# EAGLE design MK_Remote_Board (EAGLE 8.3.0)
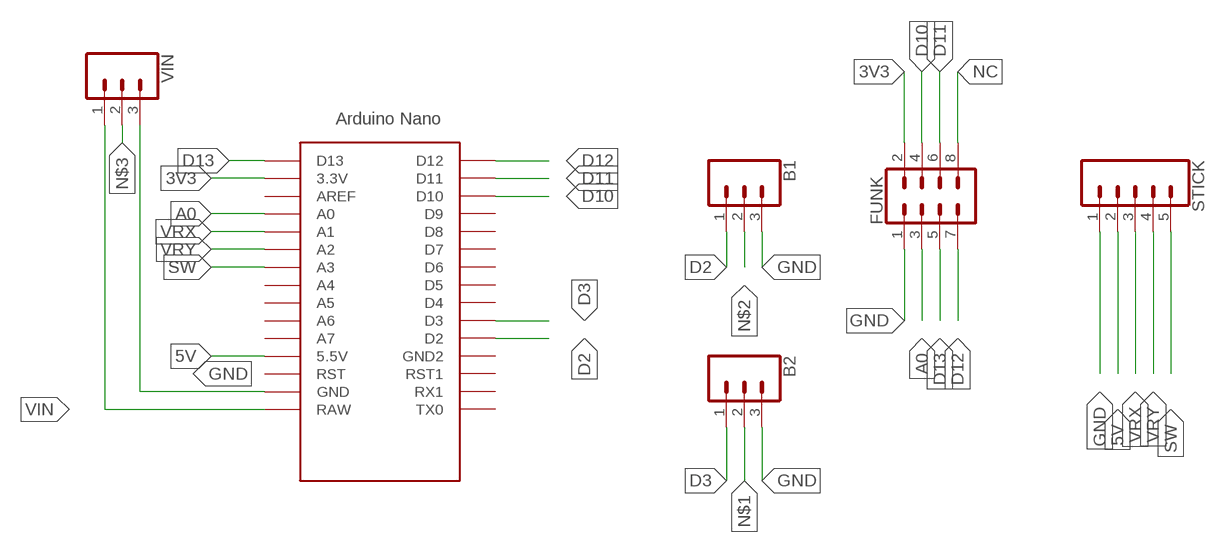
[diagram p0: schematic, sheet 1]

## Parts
B1  CONN_03  [1X03]
B2  CONN_03  [1X03]
FUNK  CONN_04X2  [2X4]
STICK  CONN_05  [1X05]
U$1  NANO  [NANO]
VIN  CONN_03  [1X03]

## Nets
3V3: FUNK.2 U$1.3.3V
5V: STICK.2 U$1.5V(5.5V)
A0: FUNK.3 U$1.A0
D2: B1.1 U$1.D2
D3: B2.1 U$1.D3
D10: FUNK.4 U$1.D10
D11: FUNK.6 U$1.D11
D12: FUNK.7 U$1.D12
D13: FUNK.5 U$1.D13
GND: B1.3 B2.3 FUNK.1 STICK.1 U$1.GND VIN.3
N$1: B2.2
N$2: B1.2
N$3: VIN.2
NC: FUNK.8
SW: STICK.5 U$1.A3
VIN: U$1.RAW VIN.1
VRX: STICK.3 U$1.A1
VRY: STICK.4 U$1.A2
Unconnected: U$1.A4 U$1.A5 U$1.A6 U$1.A7 U$1.AREF U$1.D4 U$1.D5 U$1.D6 U$1.D7 U$1.D8 U$1.D9 U$1.GND1(GND2) U$1.ICSP1 U$1.ICSP2 U$1.ICSP3 U$1.ICSP4 U$1.ICSP5 U$1.ICSP6 U$1.RST U$1.RST1 U$1.RX1 U$1.TX0

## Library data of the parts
B1 B2 VIN = SparkFun-Connectors:CONN_03: Multi connection point. Often used as Generic Header-pin footprint for 0.1 inch spaced/style header connections On any of the 0.1 inch spaced packages, you can populate with these: Break Away Headers - Straight (PRT-00116) Break Away Male Headers - Right Angle (PRT-00553) Female Headers (PRT-00115)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
FUNK = SparkFun-Connectors:CONN_04X2: Multi connection point. Often used as Generic Header-pin footprint for 0.1 inch spaced/style header connections On any of the 0.1 inch spaced packages, you can populate with these: Break Away Headers - Straight (PRT-00116) Break Away Male Headers - Right Angle (PRT-00553) Female Headers (PRT-00115)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
STICK = SparkFun-Connectors:CONN_05: Multi connection point. Often used as Generic Header-pin footprint for 0.1 inch spaced/style header connections On any of the 0.1 inch spaced packages, you can populate with these: Break Away Headers - Straight (PRT-00116) Break Away Male Headers - Right Angle (PRT-00553) Female Headers (PRT-00115)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
U$1 = Arduino-clone:NANO: Arduino Nano

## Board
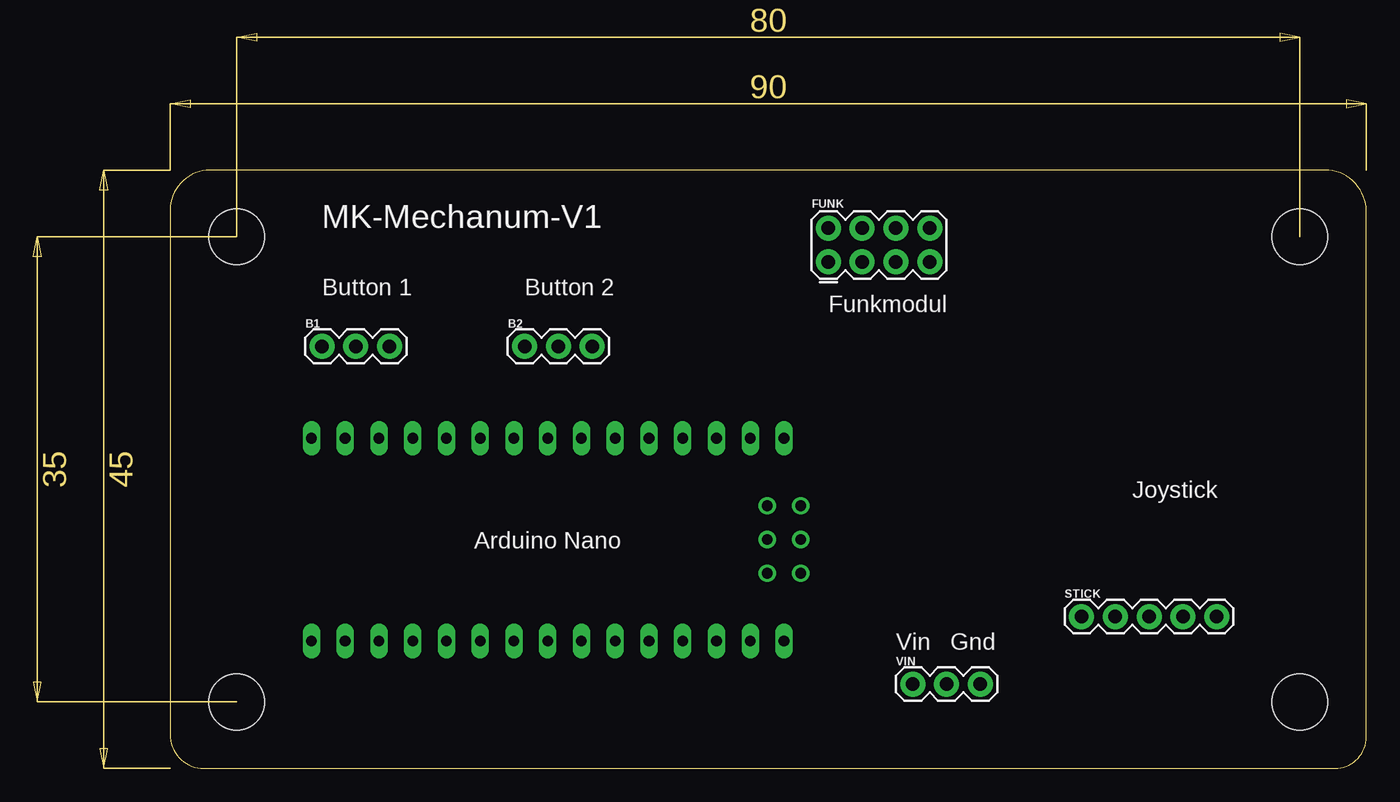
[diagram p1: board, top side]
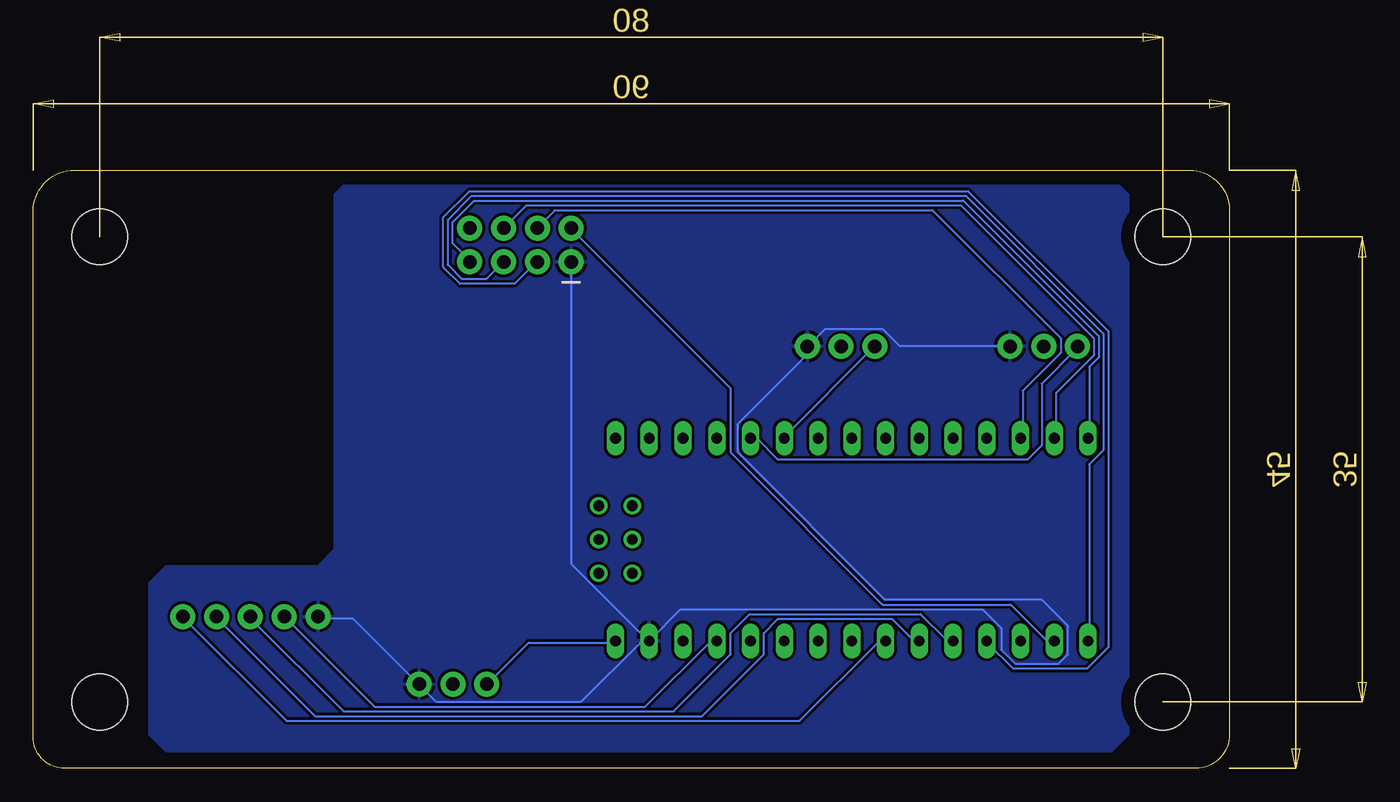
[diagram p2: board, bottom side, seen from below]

Size 100.3 x 55.3 mm. Coordinates in mm from the lower left corner, seen from the top.
Outline: 97.21,45 13.3,45 arc90 10.3,42 10.3,2.54 arc90 12.84,0 97.93,0 arc90 100.3,2.37 100.3,41.91 arc90 97.21,45
Copper layers (1*16): Top 0.035mm / dielectric 1.5mm / Bottom 0.035mm
Design rules "PCBway": minimum track width 6mil, minimum drill 0.3mm, track to track 0.205mm, track to pad 0.205mm, pad to pad 0.205mm, via to via 0.205mm, smd to smd 8mil, copper to edge 40mil, drill to drill 8mil, minimum pad ring 10mil, minimum via ring 8mil, stop-mask expansion 4mil, vias tented up to drill 25mil, thermal gap 10mil
Holes 4.2 mm at 15.3,40 15.3,5 95.3,40 95.3,5

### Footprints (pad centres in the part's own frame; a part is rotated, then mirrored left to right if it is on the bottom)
1X03 = drill 1.016 pad 1.88: 1 0,0; 2 2.54,0; 3 5.08,0
2X4 = drill 1.016 pad 1.88: 1 -3.81,-1.27; 2 -3.81,1.27; 3 -1.27,-1.27; 4 -1.27,1.27; 5 1.27,-1.27; 6 1.27,1.27; 7 3.81,-1.27; 8 3.81,1.27
1X05 = drill 1.016 pad 1.88: 1 0,0; 2 2.54,0; 3 5.08,0; 4 7.62,0; 5 10.16,0
NANO = drill 0.8 long: 3.3V -10.16,24.13; 5V -10.16,-1.27; A0 -10.16,19.05; A1 -10.16,16.51; A2 -10.16,13.97; A3 -10.16,11.43; A4 -10.16,8.89; A5 -10.16,6.35; A6 -10.16,3.81; A7 -10.16,1.27; AREF -10.16,21.59; D2 5.08,1.27; D3 5.08,3.81; D4 5.08,6.35; D5 5.08,8.89; D6 5.08,11.43; D7 5.08,13.97; D8 5.08,16.51; D9 5.08,19.05; D10 5.08,21.59; D11 5.08,24.13; D12 5.08,26.67; D13 -10.16,26.67; GND -10.16,-6.35; GND1 5.08,-1.27; RAW -10.16,-8.89; RST -10.16,-3.81; RST1 5.08,-3.81; RX1 5.08,-6.35; TX0 5.08,-8.89 | drill 0.8: ICSP1 -5.08,-10.16; ICSP2 -5.08,-7.62; ICSP3 -2.54,-10.16; ICSP4 -2.54,-7.62; ICSP5 0,-10.16; ICSP6 0,-7.62

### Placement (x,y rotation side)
B1  21.73,31.75 0 top
B2  36.97,31.75 0 top
FUNK  63.64,39.37 0 top
STICK  78.88,11.43 0 top
U$1  47.6,19.76 90 top
VIN  66.18,6.35 0 top

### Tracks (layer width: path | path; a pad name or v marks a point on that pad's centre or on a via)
3V3
  Bottom 0.152: U$1.3.3V 23.52,9.65 24.06,9.65 26.74,12.33 36.39,12.33 47.83,23.77 47.83,28.59 59.8,40.56 FUNK.2
5V
  Bottom 0.152: U$1.5V 48.9,9.47 49.44,9.47 54.26,4.65 74.63,4.65 81.24,11.26 STICK.2
A0
  Bottom 0.152: U$1.A0 28.53,9.47 26.56,7.5 21.02,7.5 19.41,9.11 19.41,32.88 29.96,43.42 67.48,43.42 69.45,41.46 69.45,37.71 68.2,36.45 64.09,36.45 62.48,38.06 FUNK.3
D2
  Bottom 0.152: U$1.D2 46.22,24.84 45.86,24.84 44.25,23.23 25.49,23.23 24.42,24.3 24.42,28.95 21.74,31.63 B1.1
D3
  Bottom 0.152: U$1.D3 43.72,25.02 37.11,31.63 B2.1
D10
  Bottom 0.152: U$1.D10 25.85,25.02 25.85,28.41 22.99,31.27 22.99,32.34 32.64,41.99 61.05,41.99 62.3,40.74 FUNK.4
D11
  Bottom 0.152: U$1.D11 23.34,25.02 23.34,28.23 20.49,31.09 20.49,32.34 30.49,42.35 63.2,42.35 64.8,40.74 FUNK.6
D12
  Bottom 0.152: U$1.D12 20.84,25.02 20.84,30.2 20.13,30.91 20.13,32.52 30.31,42.71 67.13,42.71 68.73,41.1 68.73,39.49 67.48,38.24 FUNK.7
D13
  Bottom 0.152: U$1.D13 20.84,9.65 20.84,22.87 19.77,23.95 19.77,32.7 30.14,43.07 67.31,43.07 69.09,41.28 69.09,37.88 68.02,36.81 66.23,36.81 64.98,38.06 FUNK.5
GND
  Bottom 0.152: B1.3 26.92,31.81 35.14,31.81 36.39,33.06 40.68,33.06 41.93,31.81 B2.3 42.11,31.63 42.11,31.09 47.29,25.91 47.29,23.77 36.21,12.69 24.42,12.69 22.45,10.72 22.45,8.58 23.17,7.86 26.38,7.86 27.46,8.94 27.46,10.54 28.89,11.97 51.58,11.97 53.9,9.65 U$1.GND | U$1.GND 54.08,9.47 54.62,9.47 59.08,5 69.99,5 71.24,6.25 VIN.3 71.42,6.43 76.24,11.26 78.74,11.26 STICK.1 | FUNK.1 59.8,38.06 59.8,15.37 54.08,9.65 U$1.GND
  pour Bottom (isolate 0): 17.92,2.54 19.19,1.27 90.31,1.27 91.58,2.54 91.58,13.97 90.31,15.24 78.88,15.24 77.61,16.51 77.61,43.18 76.34,44.45 19.19,44.45 17.92,43.18
SW
  Bottom 0.152: U$1.A3 36.21,9.47 36.75,9.47 42.64,3.57 81.24,3.57 88.93,11.26 STICK.5
VIN
  Bottom 0.152: U$1.RAW 56.58,9.47 63.02,9.47 66.05,6.43 VIN.1
VRX
  Bottom 0.152: U$1.A1 31.21,9.65 31.57,9.65 33.53,11.62 46.4,11.62 47.83,10.19 47.83,8.58 52.12,4.29 76.95,4.29 83.92,11.26 STICK.3
VRY
  Bottom 0.152: U$1.A2 33.71,9.65 34.07,9.65 35.67,11.26 44.25,11.26 45.33,10.19 45.33,8.58 49.97,3.93 79.1,3.93 86.43,11.26 STICK.4

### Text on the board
tNames: MK-Mechanum-V1 | Button 1 | Button 2 | Funkmodul | Joystick | Arduino Nano | Vin Gnd

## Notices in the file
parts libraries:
SparkFun-Connectors: Licensing: Creative Commons ShareAlike 4.0 International - https://creativecommons.org/licenses/by-sa/4.0
